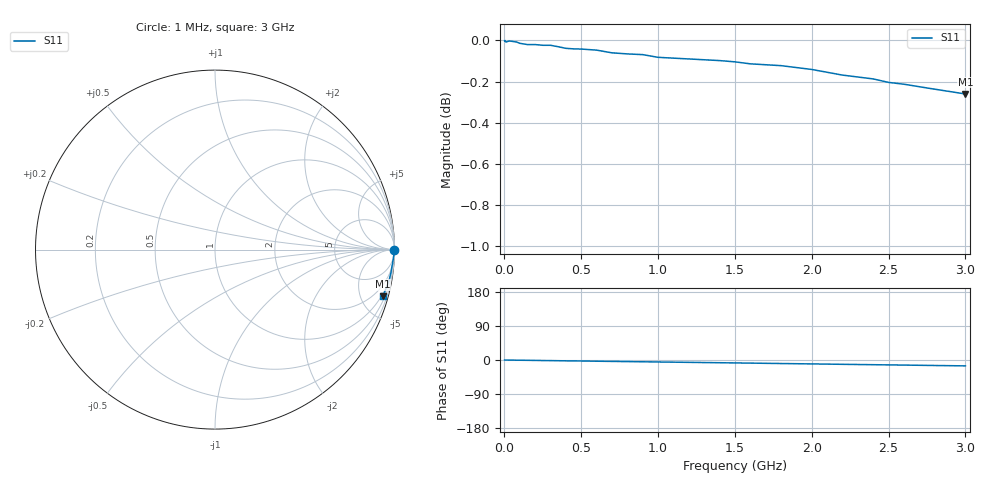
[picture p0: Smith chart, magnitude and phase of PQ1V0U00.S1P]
! SIEMENS Small Signal Semiconductors
! BAR64-04
! Si PIN Diode in SOT23 (2 diodes in series, pin 3 open)
! VR = 1 V
! S-Parameters:  July  1992
# GHz  S  MA  R  50
!  f  S11
! GHz  MAG  ANG
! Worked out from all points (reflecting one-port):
!   33 points, 1 MHz to 3 GHz, reference 50 ohm
!   lowest |S11| = -0.3 dB at 3 GHz (marker M1), VSWR 66.80, Z = 40.7 - j363 ohm
!   phase of S11 starts at 0 deg and turns -16 deg over the sweep
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0.001  0.9998 0.0
0.003  1 0.0
0.01  0.9991 -0.1
0.03  0.9997 -0.2
0.05  0.9995 -0.3
0.06  0.9994 -0.4
0.1  0.9984 -0.6
0.15  0.9977 -0.8
0.25  0.9973 -1.4
0.3  0.9973 -1.6
0.4  0.9956 -2.2
0.5  0.9952 -2.6
0.6  0.9946 -3.2
0.7  0.9931 -3.7
0.8  0.9925 -4.2
0.9  0.9921 -4.7
1  0.9906 -5.2
1.2  0.9897 -6.2
1.4  0.9888 -7.2
1.6  0.987 -8.2
1.8  0.986 -9.3
2  0.9839 -10.3
2.2  0.9808 -11.4
2.4  0.9787 -12.4
2.5  0.9768 -12.9
2.6  0.9758 -13.4
2.8  0.9731 -14.5
3  0.9705 -15.5
